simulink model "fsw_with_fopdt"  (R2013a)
settings: Solver=ode45  StartTime=0.0  StopTime=200  RelTol=1e-3
libraries: simulink x5, realtime_pacer_lib x1

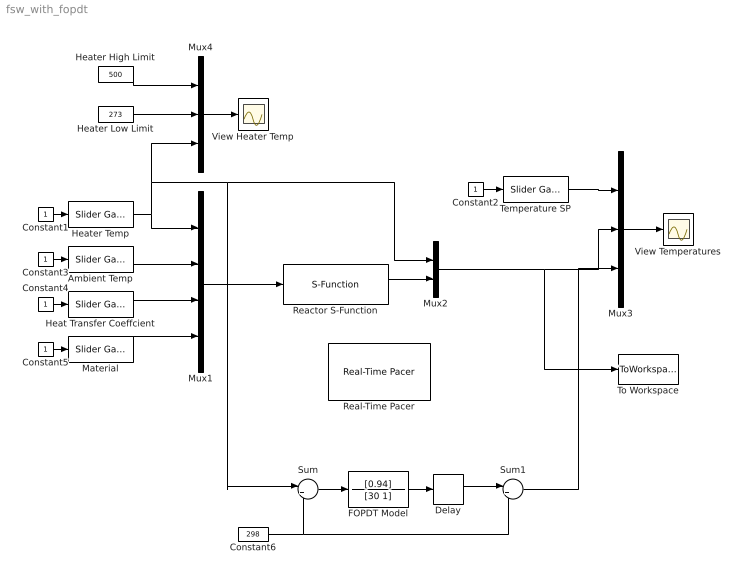
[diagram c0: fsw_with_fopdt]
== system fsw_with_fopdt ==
  Ambient Temp : simulink/Math Operations/Slider Gain  low=273  gain=300  high=320
  Constant{1..5} (5 alike) : Constant
  Constant6 : Constant  Value=298
  Delay : TransportDelay  DelayTime=5
  FOPDT Model : TransferFcn  Numerator=[0.94]  Denominator=[30 1]
  Heat Transfer Coeffcient : simulink/Math Operations/Slider Gain  low=0  gain=100  high=1000
  Heater High Limit : Constant  Value=500
  Heater Low Limit : Constant  Value=273
  Heater Temp : simulink/Math Operations/Slider Gain  low=273  gain=350  high=500
  Material : simulink/Math Operations/Slider Gain  low=0  gain=0  high=1
  Mux1 : Mux
  Mux2 : Mux  Inputs=2
  Mux3 : Mux  Inputs=3
  Mux4 : Mux  Inputs=3
  Reactor S-Function : S-Function  FunctionName=rod  EnableBusSupport=off
  Real-Time Pacer : realtime_pacer_lib/Real-Time Pacer  simTimePerRealTime=3
  Sum : Sum  Inputs=|+-
  Sum1 : Sum  Inputs=|++
  Temperature SP : simulink/Math Operations/Slider Gain  low=280  gain=380  high=400
  To Workspace : ToWorkspace  VariableName=results  SampleTime=0.5  SaveFormat=Timeseries
  View Heater Temp : Scope
  View Temperatures : Scope
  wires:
  Mux1/1 -> Reactor S-Function/1
  Constant2/1 -> Temperature SP/1
  Temperature SP/1 -> Mux3/1
  Mux3/1 -> View Temperatures/1
  Heater Temp/1 -> Sum/1, Mux2/1, Mux4/3, Mux1/1
  Heater High Limit/1 -> Mux4/1
  Heater Low Limit/1 -> Mux4/2
  Mux4/1 -> View Heater Temp/1
  Constant1/1 -> Heater Temp/1
  Constant3/1 -> Ambient Temp/1
  Ambient Temp/1 -> Mux1/2
  Constant4/1 -> Heat Transfer Coeffcient/1
  Heat Transfer Coeffcient/1 -> Mux1/3
  Constant5/1 -> Material/1
  Material/1 -> Mux1/4
  Reactor S-Function/1 -> Mux2/2
  Mux2/1 -> To Workspace/1, Mux3/2
  FOPDT Model/1 -> Delay/1
  Constant6/1 -> Sum1/2, Sum/2
  Sum/1 -> FOPDT Model/1
  Delay/1 -> Sum1/1
  Sum1/1 -> Mux3/3
